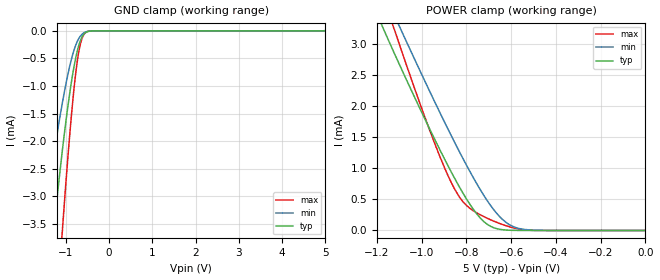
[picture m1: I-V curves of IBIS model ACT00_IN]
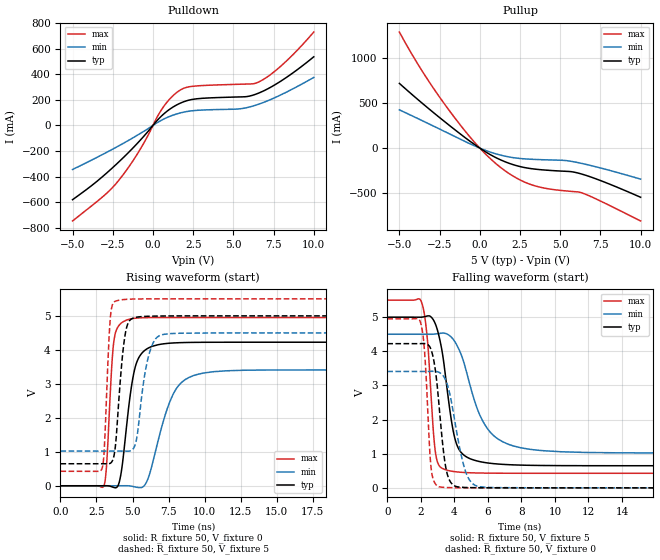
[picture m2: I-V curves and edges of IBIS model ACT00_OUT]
| TEXAS INSTRUMENTS INCORPORATED
| Standard Linear and Logic Group
| IBIS Model of SN74ACT00
| QUADRUPLE 2-INPUT POSITIVE-NAND GATES
| This file contains package information for the following:
|  SOIC 14-pin (D) package as [Component] ACT00_D
|  SSOP 14-pin (DB) package as [Component] ACT00_DB
|  PDIP 14-pin (N) package as [Component] ACT00_N
|  SOP 14-pin (NS) package as [Component] ACT00_NS
|  TSSOP 14-pin (PW) package as [Component] ACT00_PW
| This device can be powered at the following Vccs:
|  5 volt Vcc
| This file provides unique models under the [Model Selector] for each Vcc.
| For operation at a specific Vcc, select the appropriate model after each
| [Model Selector] keyword.
[IBIS Ver]   3.2
[Comment char]  |_char
[File Name]   sn74act00.ibs
[File Rev]   1.1 | x_die
[Date]   May 14, 2007
[Source]   Data created from TI-SPICE simulations at TI-SLL.
[Notes]   The following is an IBIS list for the SN74ACT00.
   Please contact sllibis@ti.com with questions and
   comments concerning SLL IBIS models.
   This IBIS model is created from a BA (back annotated
   netlist)
   - FILE REV HISTORY
   - 1.1 Release IBIS file on 08/15/07
[Disclaimer] Property of Texas Instruments Incorporated.  Unauthorized
   reproduction and/or distribution is strictly prohibited.
   This product is protected under copyright law.
   Created  2007, (C) Copyright  2007, Texas Instruments
   Incorporated, All Rights Reserved
   UNLESS THERE IS A SIGNED, WRITTEN AGREEMENT TO THE
   CONTRARY, TEXAS INSTRUMENTS (TI) IS PROVIDING THE IBIS
   MODELS  AND WITHOUT ANY WARRANTY, EXPRESSED OR
   IMPLIED.  TI assumes no liability for:
   1) the accuracy of the IBIS models provided to your
   company;
   2) the proper functioning of these IBIS Models in your
   design or for any resulting applications; or
   3) infringement of patents, copyrights or intellectual
   property rights resulting from your use of these IBIS
   models.
   TI provides IBIS Models as a service to our customers.
   You and your company shall not distribute, sell or give
   these models to anyone else without prior written
   permission from TI.
   TI reserves the right to make changes to our products or
   to discontinue any semiconductor product or service
   without notice, and advises our customers to obtain the
   latest version of relevant information to verify, before
   placing orders, that the information being relied on is
   current.
   Please be aware that your receipt and use of the IBIS
   information provided shall serve as acceptance of these
   terms and conditions.  If you do not accept these terms,
   you should return or destroy the IBIS models and any
   other accompanying information immediately.
| Component SN74ACT00_D 14-PIN SOIC
[Component]   SN74ACT00_D
[Manufacturer]   Texas Instruments, Inc.
[Package]
|   typ   min   max
R_pkg   3.100e-02   2.800e-02   3.400e-02
L_pkg   3.109e-09   2.462e-09   3.889e-09
C_pkg   4.730e-13   3.630e-13   6.280e-13
[Pin]   signal_name   model_name   R_pin   L_pin   C_pin
1   1A   ACT00_IN   3.300e-02   3.854e-09   6.220e-13
2   1B   ACT00_IN   3.200e-02   3.188e-09   4.730e-13
3   1Y   ACT00_OUT   2.800e-02   2.462e-09   3.770e-13
4   2A   ACT00_IN   3.100e-02   2.596e-09   3.630e-13
5   2B   ACT00_IN   2.800e-02   2.521e-09   3.720e-13
6   2Y   ACT00_OUT   3.400e-02   3.250e-09   4.760e-13
7   GND   GND   3.400e-02   3.889e-09   6.280e-13
8   3Y   ACT00_OUT   3.400e-02   3.889e-09   6.280e-13
9   3A   ACT00_IN   3.400e-02   3.250e-09   4.760e-13
10   3B   ACT00_IN   2.800e-02   2.521e-09   3.720e-13
11   4Y   ACT00_OUT   3.100e-02   2.596e-09   3.640e-13
12   4A   ACT00_IN   2.800e-02   2.462e-09   3.770e-13
13   4B   ACT00_IN   3.200e-02   3.188e-09   4.730e-13
14   VCC   POWER   3.300e-02   3.854e-09   6.220e-13
| Component SN74ACT00_DB 14-PIN SSOP
[Component]   SN74ACT00_DB
[Manufacturer]   Texas Instruments, Inc.
[Package]
|   typ   min   max
R_pkg   4.400e-02   4.100e-02   4.600e-02
L_pkg   3.551e-09   3.258e-09   3.927e-09
C_pkg   4.020e-13   3.600e-13   4.210e-13
[Pin]   signal_name   model_name   R_pin   L_pin   C_pin
1   1A   ACT00_IN   4.600e-02   3.927e-09   4.080e-13
2   1B   ACT00_IN   4.400e-02   3.587e-09   4.210e-13
3   1Y   ACT00_OUT   4.100e-02   3.289e-09   3.980e-13
4   2A   ACT00_IN   4.200e-02   3.258e-09   3.600e-13
5   2B   ACT00_IN   4.100e-02   3.286e-09   4.030e-13
6   2Y   ACT00_OUT   4.400e-02   3.586e-09   4.210e-13
7   GND   GND   4.600e-02   3.927e-09   4.080e-13
8   3Y   ACT00_OUT   4.600e-02   3.927e-09   4.080e-13
9   3A   ACT00_IN   4.400e-02   3.586e-09   4.210e-13
10   3B   ACT00_IN   4.100e-02   3.286e-09   4.030e-13
11   4Y   ACT00_OUT   4.300e-02   3.258e-09   3.600e-13
12   4A   ACT00_IN   4.100e-02   3.289e-09   3.980e-13
13   4B   ACT00_IN   4.400e-02   3.587e-09   4.210e-13
14   VCC   POWER   4.600e-02   3.927e-09   4.080e-13
| Component SN74ACT00_N 14-PIN PDIP
[Component]   SN74ACT00_N
[Manufacturer]   Texas Instruments, Inc.
[Package]
|   typ   min   max
R_pkg   4.500e-02   3.700e-02   6.300e-02
L_pkg   5.407e-09   3.922e-09   6.942e-09
C_pkg   3.890e-13   2.050e-13   6.040e-13
[Pin]   signal_name   model_name   R_pin   L_pin   C_pin
1   1A   ACT00_IN   6.300e-02   6.942e-09   6.040e-13
2   1B   ACT00_IN   3.700e-02   6.200e-09   4.060e-13
3   1Y   ACT00_OUT   4.200e-02   4.389e-09   3.220e-13
4   2A   ACT00_IN   3.800e-02   3.922e-09   2.050e-13
5   2B   ACT00_IN   3.900e-02   4.301e-09   2.980e-13
6   2Y   ACT00_OUT   3.800e-02   5.329e-09   3.560e-13
7   GND   GND   5.300e-02   6.510e-09   5.440e-13
8   3Y   ACT00_OUT   5.300e-02   6.437e-09   5.390e-13
9   3A   ACT00_IN   3.900e-02   5.352e-09   3.470e-13
10   3B   ACT00_IN   4.200e-02   4.473e-09   2.970e-13
11   4Y   ACT00_OUT   4.400e-02   4.326e-09   2.250e-13
12   4A   ACT00_IN   4.200e-02   4.295e-09   2.800e-13
13   4B   ACT00_IN   4.200e-02   6.318e-09   4.180e-13
14   VCC   POWER   6.100e-02   6.900e-09   6.030e-13
| Component SN74ACT00_NS 14-PIN SOP
[Component]   SN74ACT00_NS
[Manufacturer]   Texas Instruments, Inc.
[Package]
|   typ   min   max
R_pkg   4.500e-02   3.900e-02   5.400e-02
L_pkg   3.796e-09   2.561e-09   4.952e-09
C_pkg   5.280e-13   2.880e-13   7.100e-13
[Pin]   signal_name   model_name   R_pin   L_pin   C_pin
1   1A   ACT00_IN   4.700e-02   4.867e-09   7.060e-13
2   1B   ACT00_IN   5.100e-02   4.083e-09   5.920e-13
3   1Y   ACT00_OUT   4.100e-02   2.915e-09   3.760e-13
4   2A   ACT00_IN   3.900e-02   2.561e-09   2.880e-13
5   2B   ACT00_IN   4.100e-02   3.101e-09   4.300e-13
6   2Y   ACT00_OUT   4.700e-02   4.047e-09   5.890e-13
7   GND   GND   5.100e-02   4.909e-09   7.000e-13
8   3Y   ACT00_OUT   4.500e-02   4.784e-09   6.940e-13
9   3A   ACT00_IN   5.400e-02   4.176e-09   5.970e-13
10   3B   ACT00_IN   3.900e-02   3.287e-09   4.490e-13
11   4Y   ACT00_OUT   3.900e-02   2.586e-09   2.940e-13
12   4A   ACT00_IN   4.000e-02   2.802e-09   3.710e-13
13   4B   ACT00_IN   4.900e-02   4.080e-09   5.930e-13
14   VCC   POWER   5.200e-02   4.952e-09   7.100e-13
| Component SN74ACT00_PW 14-PIN TSSOP
[Component]   SN74ACT00_PW
[Manufacturer]   Texas Instruments, Inc.
[Package]
|   typ   min   max
R_pkg   3.200e-02   2.900e-02   3.500e-02
L_pkg   2.378e-09   2.170e-09   2.680e-09
C_pkg   3.140e-13   2.700e-13   3.350e-13
[Pin]   signal_name   model_name   R_pin   L_pin   C_pin
1   1A   ACT00_IN   3.300e-02   2.618e-09   3.300e-13
2   1B   ACT00_IN   3.100e-02   2.313e-09   3.170e-13
3   1Y   ACT00_OUT   3.000e-02   2.310e-09   3.140e-13
4   2A   ACT00_IN   3.100e-02   2.173e-09   2.720e-13
5   2B   ACT00_IN   3.000e-02   2.204e-09   3.090e-13
6   2Y   ACT00_OUT   3.200e-02   2.315e-09   3.170e-13
7   GND   GND   3.500e-02   2.680e-09   3.350e-13
8   3Y   ACT00_OUT   3.300e-02   2.640e-09   3.330e-13
9   3A   ACT00_IN   3.400e-02   2.347e-09   3.190e-13
10   3B   ACT00_IN   2.900e-02   2.277e-09   3.130e-13
11   4Y   ACT00_OUT   3.100e-02   2.170e-09   2.700e-13
12   4A   ACT00_IN   3.100e-02   2.244e-09   3.110e-13
13   4B   ACT00_IN   3.300e-02   2.343e-09   3.210e-13
14   VCC   POWER   3.500e-02   2.657e-09   3.320e-13
| Models and submodels in the file (2): ACT00_IN (Input), ACT00_OUT (Output)
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[Model]   ACT00_IN
Model_type  Input
Vinl=0.8
Vinh=2.0
| variable   typ   min   max
C_comp   0.80pF   0.70pF   1.27pF
[Temperature Range]   40   100   -40
| Ambient temperature   25   85   -40
[Voltage range]   5   4.5   5.5
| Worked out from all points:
|   GND clamp passes 1 mA (typ) near -0.88 V on its own axis
|   POWER clamp passes 1 mA (typ) near -0.88 V on its own axis
[GND Clamp]
| ACT00_IN
|   Voltage   I(typ)   I(min)   I(max)
-5V       -46.92mA   -30.58mA   -59.62mA
-1.56V    -6.035mA   -3.826mA   -9.528mA
-1.51V    -5.59mA    -3.537mA   -8.882mA
-1.305V   -3.869mA   -2.418mA   -6.312mA
-1.255V   -3.478mA   -2.163mA   -5.708mA
-1.08V    -2.21mA    -1.334mA   -3.692mA
-1.06V    -2.076mA   -1.247mA   -3.474mA
-900mV    -1.111mA   -628.4uA   -1.852mA
-770mV    -508.4uA   -270.1uA   -799.3uA
-670mV    -203.9uA   -108.8uA   -280.1uA
-550mV    -38.99uA   -24.34uA   -40.29uA
5V        16.38nA    4.859uA    150.6nA
[POWER Clamp]
| ACT00_IN
|   Voltage   I(typ)   I(min)   I(max)
-5V       45.74mA    45.24mA    49.64mA
-1.17V    3.235mA    3.838mA    3.746mA
-1.125V   2.87mA     3.482mA    3.262mA
-1.075V   2.477mA    3.09mA     2.732mA
-965mV    1.638mA    2.244mA    1.62mA
-895mV    1.129mA    1.722mA    985.3uA
-840mV    755.6uA    1.327mA    587.5uA
-785mV    423.6uA    951.8uA    357.6uA
-695mV    72.53uA    417uA      176.8uA
-640mV    12.79uA    181.6uA    97.2uA
-585mV    1.851uA    53.91uA    37.94uA
-84.45fV  16.38nA    947.5pA    229.7nA
[Model]   ACT00_OUT
Model_type  Output
Vref =   0
Rref =   500
Cref =   50p
Vmeas =   1.5
| variable   typ   min   max
C_comp   12.06pF   5.64pF   19.76pF
| C_pullup   13.15pF   5.64pF   19.76pF
| C_pulldown   10.97pF   6.03pF   16.51pF
[Temperature Range]   40   100   -40
| Ambient temperature   25   85   -40
[Voltage range]   5   4.5   5.5
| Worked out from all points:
|   slope of the pulldown table from 0 to 0.75 V, typ, clamps not added: 7.64 ohm
|   slope of the pullup table from 0 to 0.75 V, typ, clamps not added: 9.15 ohm
|   rising waveform, R_fixture 50, V_fixture 0: 20-80 % time 766ps typ, 1.46ns min, 379ps max; typ from 0 V to 4.22 V
|   falling waveform, R_fixture 50, V_fixture 5: 20-80 % time 776ps typ, 1.52ns min, 421ps max; typ from 5 V to 0.648 V
|   rising waveform, R_fixture 50, V_fixture 5: 20-80 % time 498ps typ, 711ps min, 307ps max; typ from 0.648 V to 5 V
|   falling waveform, R_fixture 50, V_fixture 0: 20-80 % time 525ps typ, 809ps min, 317ps max; typ from 4.22 V to 0 V
[Pulldown]
| ACT00_OUT
|   Voltage   I(typ)   I(min)   I(max)
-5V       -580.4mA   -344.3mA   -746.8mA
-3V       -385.5mA   -218.2mA   -544mA
-2.135V   -286.7mA   -160.2mA   -430.5mA
-865mV    -125.8mA   -68.55mA   -201.6mA
555mV     76.37mA    42.29mA    127mA
1.47V     159.9mA    89.76mA    256.7mA
1.91V     184.9mA    104mA      290.3mA
2.405V    202.4mA    114.2mA    305.1mA
5.375V    222.9mA    129.7mA    322mA
6.535V    250.9mA    164.4mA    337.7mA
8.035V    353.1mA    244mA      472.8mA
10V       536.5mA    375.2mA    730.1mA
[Pullup]
| ACT00_OUT
|   Voltage   I(typ)   I(min)   I(max)
-5V       714.7mA    422.3mA    1.282A
-3.495V   482.8mA    295.7mA    826.6mA
-1.81V    239.1mA    150.5mA    393.9mA
-145mV    17.72mA    11.1mA     28.11mA
570mV     -63.95mA   -39.32mA   -102.7mA
1.285V    -129.4mA   -77.34mA   -212.7mA
2.305V    -195.1mA   -111mA     -333.4mA
3.33V     -230.3mA   -124.6mA   -411.9mA
5.235V    -255.6mA   -135.9mA   -471.4mA
6.175V    -279mA     -163.2mA   -486.7mA
7.215V    -339.4mA   -206.5mA   -560.8mA
10V       -543.6mA   -343.1mA   -805.8mA
[Ramp]
| ACT00_OUT
| variable   typ   min   max
dV/dt_r   2.57/7.74E-10   2.08/1.47E-09   3.00/3.86E-10
dV/dt_f   2.63/7.88E-10   2.11/1.53E-09   3.07/4.32E-10
R_load = 50
[Rising Waveform]
| ACT00_OUT
R_fixture =   50
C_fixture =   0
L_fixture =   0
V_fixture =   0
V_fixture_min = 0
V_fixture_max = 0
|   Time   V(typ)   V(min)   V(max)
0s        1.105nV    1.752nV    706.6pV
3.01ns    279.9uV    7.32uV     -10.28mV
3.2ns     655.7uV    7.505uV    607.2mV
3.72ns    -52.63mV   9.977uV    4.298V
4.185ns   315.7mV    170.1uV    4.774V
4.805ns   2.554V     -4.018mV   4.903V
5.875ns   3.993V     35.44mV    4.946V
7.86ns    4.203V     2.728V     4.951V
9.935ns   4.222V     3.318V     4.951V
50ns      4.224V     3.41V      4.951V
[Falling Waveform]
| ACT00_OUT
R_fixture =   50
C_fixture =   0
L_fixture =   0
V_fixture =   5
V_fixture_min = 4.5
V_fixture_max = 5.5
|   Time   V(typ)   V(min)   V(max)
0s        5V         4.5V       5.5V
2.05ns    5.001V     4.5V       5.428V
2.39ns    5.036V     4.499V     4.343V
2.89ns    4.771V     4.509V     975.4mV
3.27ns    3.991V     4.533V     572mV
3.705ns   2.368V     4.463V     500.3mV
4.305ns   1.102V     4.021V     459.8mV
5.93ns    732.9mV    1.765V     431.5mV
8.365ns   661.4mV    1.139V     426.8mV
50ns      647.6mV    1.02V      426.5mV
[Rising Waveform]
| ACT00_OUT
R_fixture =   50
C_fixture =   0
L_fixture =   0
V_fixture =   5
V_fixture_min = 4.5
V_fixture_max = 5.5
|   Time   V(typ)   V(min)   V(max)
0s        647.6mV    1.02V      426.5mV
2.89ns    647.7mV    1.02V      516.5mV
3.045ns   647.6mV    1.02V      1.117V
3.475ns   666.8mV    1.02V      5.001V
4.02ns    2.337V     1.02V      5.457V
4.705ns   4.796V     1.019V     5.489V
5.25ns    4.957V     1.311V     5.497V
6.19ns    4.989V     3.931V     5.5V
7.19ns    4.996V     4.457V     5.5V
50ns      5V         4.5V       5.5V
[Falling Waveform]
| ACT00_OUT
R_fixture =   50
C_fixture =   0
L_fixture =   0
V_fixture =   0
V_fixture_min = 0
V_fixture_max = 0
|   Time   V(typ)   V(min)   V(max)
0s        4.224V     3.41V      4.951V
1.98ns    4.225V     3.41V      4.846V
2.23ns    4.227V     3.41V      3.935V
2.615ns   4.04V      3.413V     570.2mV
3.145ns   2.082V     3.368V     24.39mV
3.435ns   751.2mV    3.202V     12.06mV
3.72ns    212.9mV    2.764V     6.939mV
4.64ns    11.65mV    520.1mV    1.714mV
5.5ns     3.595mV    33.39mV    557.4uV
50ns      -3.185nV   -4.765nV   -7.072nV
